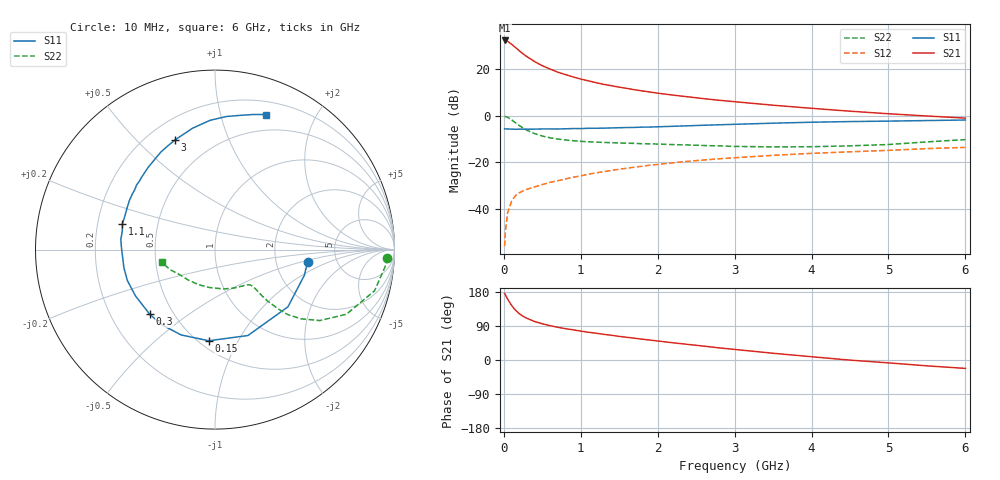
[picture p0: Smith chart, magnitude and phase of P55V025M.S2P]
! SIEMENS Small Signal Semiconductors
! BFP183
! Si NPN RF Bipolar Junction Transistor in SOT143
! VCE = 5 V  IC = 25 mA
! Common Emitter S-Parameters:  March  1996
# GHz  S  MA  R  50
!  f  S11  S21  S12  S22
! GHz  MAG  ANG  MAG  ANG  MAG  ANG  MAG  ANG
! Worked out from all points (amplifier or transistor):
!   36 points, 10 MHz to 6 GHz, reference 50 ohm
!   highest |S21| = 32.2 dB at 10 MHz (marker M1)
!   |S21| within 3 dB of that: start of sweep to 150.8 MHz
!   unconditionally stable (mu >= 1): 774.1 MHz to 5.669 GHz
!   at 250 MHz: K = 0.52, MSG = 29.3 dB, |S12| = -32.3 dB
!   at 1.4 GHz: K = 1.13, MAG = 15.9 dB, |S12| = -23.5 dB
!   at 6 GHz: K = 0.97, MSG = 6.3 dB, |S12| = -13.6 dB
!   S11 on the Smith chart (normalised r, x): 10 MHz: 3.06, -0.56; 150 MHz: 0.56, -0.76; 300 MHz: 0.37, -0.36; 1.1 GHz: 0.31, +0.12; 3 GHz: 0.31, +0.65; 6 GHz: 0.33, +1.39
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0.01  0.5206 -7.4  40.6 175.6  0.0016 87.0  0.9612 -2.7
0.02  0.5181 -16.0  40.47 172.1  0.0033 76.2  0.9525 -5.8
0.05  0.5165 -38.1  38.79 160.4  0.0084 79.0  0.9179 -14.5
0.1  0.5127 -69.0  33.71 144.3  0.0146 64.7  0.8158 -26.2
0.15  0.509 -93.9  28.82 131.7  0.0193 57.1  0.7053 -34.1
0.2  0.5116 -111.7  24.5 122.4  0.0222 53.9  0.6136 -38.9
0.25  0.5127 -125.0  20.96 115.3  0.0244 50.9  0.5428 -41.8
0.3  0.5119 -135.3  18.28 110.0  0.0264 50.4  0.486 -43.1
0.4  0.5127 -149.9  14.35 101.5  0.0297 50.3  0.4113 -44.4
0.5  0.5178 -160.6  11.68 95.6  0.0333 50.6  0.3647 -44.5
0.6  0.5175 -168.7  9.941 90.6  0.0372 52.1  0.3351 -44.3
0.7  0.5166 -175.8  8.51 86.4  0.0402 53.8  0.3143 -44.1
0.8  0.5215 178.6  7.546 82.7  0.0439 53.7  0.3003 -44.1
1  0.5269 168.5  6.049 76.2  0.0511 54.7  0.2812 -44.9
1.1  0.5352 164.5  5.535 73.2  0.0556 54.9  0.2749 -45.6
1.5  0.5499 150.1  4.06 62.3  0.0712 53.9  0.2593 -49.9
2.2  0.5899 129.3  2.744 45.4  0.0977 49.3  0.2392 -62.8
3  0.6504 110.0  1.981 27.9  0.1251 42.2  0.2187 -83.1
3.5  0.6877 100.5  1.668 17.8  0.1408 37.8  0.2135 -98.1
4.5  0.7446 85.0  1.242 -0.3  0.1676 28.5  0.2251 -130.7
5.5  0.7827 74.1  0.98 -15.4  0.1964 20.8  0.2734 -155.9
6  0.804 69.4  0.883 -22.2  0.2086 16.1  0.3061 -166.6
